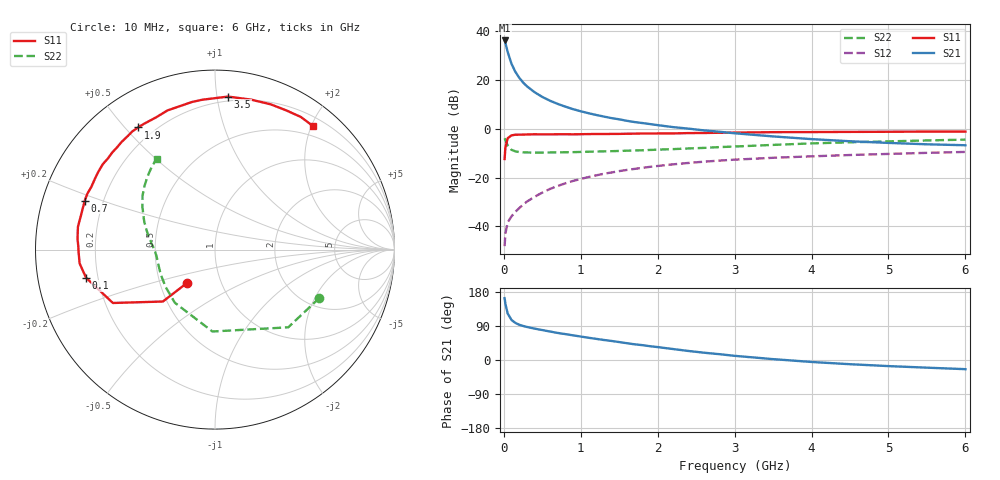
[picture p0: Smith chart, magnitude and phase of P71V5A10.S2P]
! SIEMENS Small Signal Semiconductors
! BFP196
! Si NPN RF Bipolar Junction Transistor in SOT143
! VCE = 1.5 V  IC = 100 mA
! Common Emitter S-Parameters:  May  1996
# GHz  S  MA  R  50
!  f  S11  S21  S12  S22
! GHz  MAG  ANG  MAG  ANG  MAG  ANG  MAG  ANG
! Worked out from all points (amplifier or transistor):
!   36 points, 10 MHz to 6 GHz, reference 50 ohm
!   highest |S21| = 36.3 dB at 10 MHz (marker M1)
!   |S21| within 3 dB of that: start of sweep to 36.18 MHz
!   unconditionally stable (mu >= 1): start of sweep to 11.19 MHz; 216.4 MHz to end of sweep
!   at 250 MHz: K = 1.04, MAG = 23.8 dB, |S12| = -31.2 dB
!   at 1.4 GHz: K = 1.14, MAG = 8.9 dB, |S12| = -17.9 dB
!   at 6 GHz: K = 1.03, MAG = 0.2 dB, |S12| = -9.5 dB
!   S11 on the Smith chart (normalised r, x): 10 MHz: 0.69, -0.27; 100 MHz: 0.15, -0.11; 700 MHz: 0.13, +0.18; 1.9 GHz: 0.14, +0.54; 3.5 GHz: 0.17, +1.08; 6 GHz: 0.34, +2.03
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0.01  0.2404 -129.9  65.43 163.2  0.0039 67.3  0.6413 -24.8
0.02  0.4099 -135.1  58.47 148.3  0.0071 61.6  0.595 -46.7
0.05  0.6419 -152.4  37.97 122.5  0.012 51.4  0.4565 -91.8
0.1  0.7354 -167.7  21.6 105.5  0.016 51.1  0.3711 -127.1
0.15  0.7582 -174.2  14.82 97.9  0.0198 54.7  0.3449 -142.9
0.2  0.76 -178.7  11.22 93.0  0.0236 59.0  0.3343 -151.9
0.25  0.7625 178.2  8.962 89.8  0.0277 61.9  0.3302 -157.9
0.3  0.7681 175.7  7.497 87.2  0.0321 63.8  0.3275 -161.5
0.4  0.7742 170.6  5.657 82.8  0.0403 66.1  0.3263 -166.8
0.5  0.7712 167.3  4.527 79.0  0.0491 67.0  0.3263 -170.2
0.6  0.7714 163.2  3.787 75.1  0.0584 66.8  0.3272 -172.6
0.7  0.7753 159.4  3.258 71.4  0.0672 66.4  0.3287 -174.5
0.9  0.7725 153.0  2.541 65.1  0.0853 64.5  0.3327 -177.6
1.1  0.7815 146.3  2.098 58.7  0.1024 62.2  0.3392 179.9
1.4  0.7875 136.7  1.664 50.3  0.1272 57.6  0.3482 176.5
1.9  0.8041 122.2  1.255 36.4  0.166 49.6  0.369 171.0
2.2  0.8064 114.2  1.087 28.9  0.1868 44.8  0.3837 167.1
2.6  0.8229 103.7  0.931 19.3  0.2119 38.3  0.4067 161.6
3.5  0.8557 85.1  0.7 2.3  0.2548 24.9  0.4688 149.6
4.5  0.8669 69.0  0.557 -11.1  0.2905 12.6  0.5302 137.7
5.5  0.8802 57.1  0.482 -20.2  0.3217 1.6  0.5785 127.8
6  0.8786 51.5  0.461 -24.2  0.3362 -4.2  0.6016 122.8
